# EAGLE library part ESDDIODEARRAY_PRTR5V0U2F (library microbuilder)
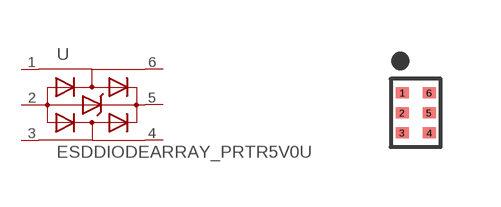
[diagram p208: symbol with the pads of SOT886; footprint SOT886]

Designator prefix U

## ESDDIODEARRAY_PRTR5V0U2F  [SOT886]
1  I/O1_1  pas
2  GND  pas
3  I/O2_1  pas
4  I/O2_2  pas
5  VBUS  pas
6  I/O1_2  pas

## Footprint SOT886 (pad centres in mm)
SOT-886 Source: PRTR5V0U2F
smd 0.325 x 0.27: 1 -0.338,0.5; 2 -0.338,0; 3 -0.338,-0.5; 4 0.338,-0.5; 5 0.338,0; 6 0.338,0.5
